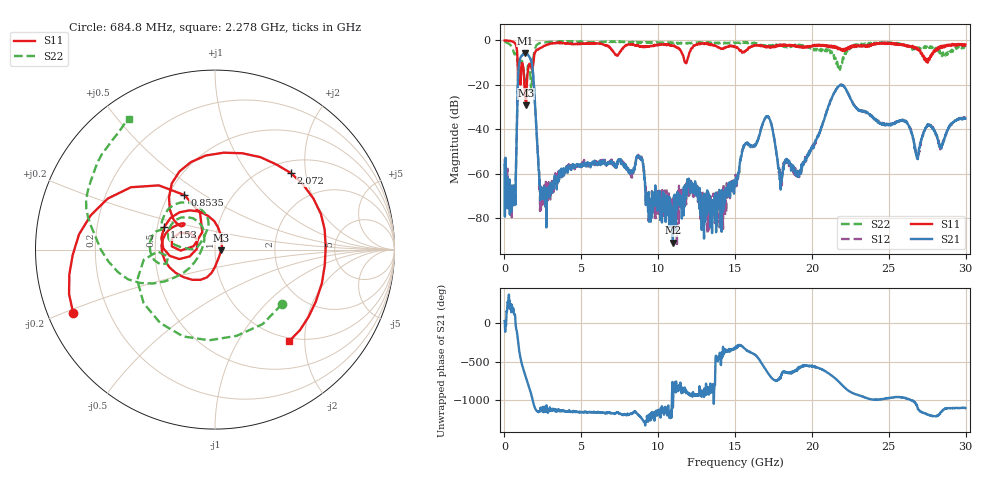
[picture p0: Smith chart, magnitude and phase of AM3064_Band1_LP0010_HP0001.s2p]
# Hz S DB R 50.0
!freq dBS11 angS11 dBS21 angS21 dBS12 angS12 dBS22 angS22
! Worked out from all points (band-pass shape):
!   1600 points, 10 MHz to 29.98 GHz, reference 50 ohm
!   highest |S21| = -5.61 dB at 1.36 GHz (marker M1); lowest = -91.1 dB at 10.96 GHz (marker M2)
!   |S21| within 3 dB of the highest: 1.007 GHz to 1.711 GHz (704.3 MHz wide, 51.8 % of centre)
!   lowest |S11| = -29.2 dB at 1.397 GHz (marker M3), VSWR 1.07, Z = 53.5 - j0.515 ohm
!   |S11| at or under -10 dB: 857.4 MHz to 1.877 GHz (1.02 GHz wide, 74.6 % of centre); 11.76 GHz to 11.84 GHz (87.94 MHz wide, 0.745 % of centre); 27.52471 GHz to 27.5297 GHz (4.982 MHz wide, 0.0181 % of centre)
!   |S22| runs from -22.8 to -0.3 dB; largest |S21 - S12| = 0.0064
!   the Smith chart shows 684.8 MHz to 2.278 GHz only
!   S11 on the Smith chart (normalised r, x): 684.8 MHz: 0.08, -0.21; 853.5 MHz: 0.60, +0.42; 1.153 GHz: 0.54, +0.15; 2.072 GHz: 1.24, +1.66; 2.278 GHz: 0.94, -1.69
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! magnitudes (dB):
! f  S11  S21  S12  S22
! 10 MHz  0.0  -56.0  -53.3  -0.3
! 684.8 MHz  -1.3  -72.2  -68.5  -6.3
! 853.5 MHz  -9.2  -22.7  -22.6  -9.9
! 1.153 GHz  -10.2  -6.8  -6.7  -9.4
! 1.36 GHz  -26.4  -5.6  -5.6  -20.9
! 1.397 GHz  -29.2  -5.7  -5.6  -19.2
! 1.772 GHz  -12.8  -10.1  -10.0  -20.4
! 2.072 GHz  -4.4  -38.9  -39.1  -2.3
! 2.278 GHz  -3.7  -65.0  -67.8  -1.2
! 5.015 GHz  -1.5  -55.9  -56.6  -0.6
! 8.763 GHz  -2.7  -52.4  -52.4  -1.0
! 9.419 GHz  -2.7  -73.7  -71.9  -1.0
! 10 GHz  -2.0  -68.3  -67.3  -0.9
! 10.96 GHz  -2.3  -91.1  -74.4  -1.1
! 15 GHz  -3.0  -65.7  -63.9  -1.2
! 17.05 GHz  -2.8  -34.3  -34.2  -2.8
! 17.97 GHz  -2.5  -67.3  -64.3  -2.0
! 19.99 GHz  -2.8  -47.9  -48.8  -3.4
! 21.85 GHz  -3.6  -20.2  -19.9  -12.5
! 25 GHz  -1.1  -37.9  -37.8  -1.2
! 26.85 GHz  -4.2  -53.3  -52.2  -3.2
! 29.98 GHz  -1.8  -35.2  -34.9  -3.1
